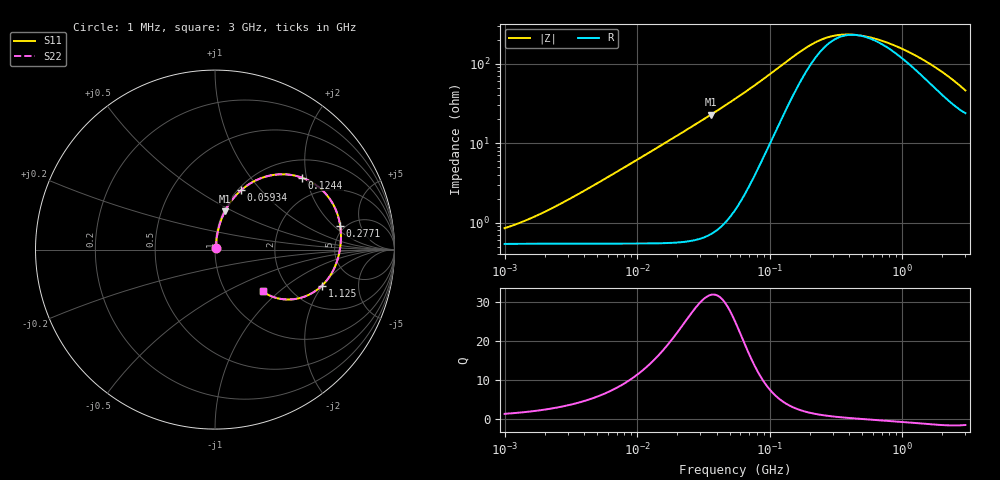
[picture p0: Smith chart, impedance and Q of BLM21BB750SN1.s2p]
! BLM21BB750SN1
# Hz S RI R 50
!Freq.(Hz) S11(Real) S11(Imag) S21(Real) S21(Imag) S12(Real) S12(Imag) S22(Real) S22(Imag)
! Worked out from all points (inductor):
!   401 points, 1 MHz to 3 GHz, reference 50 ohm
!   read as one part in series: L = 98.2 nH near 2.667 MHz
!   highest Q = 31.8 at 35.98 MHz (marker M1), where L = 101 nH
!   self-resonance near 452.7 MHz
!   S11 on the Smith chart (normalised r, x): 1 MHz: 1.01, +0.01; 59.34 MHz: 1.04, +0.78; 124.4 MHz: 1.42, +1.88; 277.1 MHz: 4.55, +2.43; 1.125 GHz: 2.97, -1.97; 3 GHz: 1.48, -0.79
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1000000  0.00541 0.00651  0.9946 -0.00651  0.9946 -0.00651  0.00541 0.00651
1786863  0.00552 0.0111  0.9945 -0.0111  0.9945 -0.0111  0.00552 0.0111
3823119  0.00595 0.0233  0.994 -0.0233  0.994 -0.0233  0.00595 0.0233
1.461624e7  0.0134 0.0884  0.9866 -0.0884  0.9866 -0.0884  0.0134 0.0884
2.362996e7  0.0265 0.1421  0.9735 -0.1421  0.9735 -0.1421  0.0265 0.1421
3.597591e7  0.0552 0.2132  0.9448 -0.2132  0.9448 -0.2132  0.0552 0.2132
5.477226e7  0.1237 0.3099  0.8763 -0.3099  0.8763 -0.3099  0.1237 0.3099
5.933785e7  0.1446 0.3299  0.8554 -0.3299  0.8554 -0.3299  0.1446 0.3299
7.248696e7  0.2118 0.3775  0.7882 -0.3775  0.7882 -0.3775  0.2118 0.3775
9.034013e7  0.3123 0.4138  0.6877 -0.4138  0.6877 -0.4138  0.3123 0.4138
1.244416e8  0.4853 0.4006  0.5147 -0.4006  0.5147 -0.4006  0.4853 0.4006
1.614254e8  0.6021 0.3268  0.3979 -0.3268  0.3979 -0.3268  0.6021 0.3268
2.094008e8  0.6695 0.2296  0.3305 -0.2296  0.3305 -0.2296  0.6695 0.2296
2.771263e8  0.6977 0.1325  0.3023 -0.1325  0.3023 -0.1325  0.6977 0.1325
3.523638e8  0.7018 0.0627  0.2982 -0.0627  0.2982 -0.0627  0.7018 0.0627
4.480278e8  0.6962 0.00245  0.3038 -0.00245  0.3038 -0.00245  0.6962 0.00245
5.929311e8  0.6809 -0.0616  0.3191 0.0616  0.3191 0.0616  0.6809 -0.0616
8.005644e8  0.6522 -0.1278  0.3478 0.1278  0.3478 0.1278  0.6522 -0.1278
1.125055e9  0.5964 -0.2004  0.4036 0.2004  0.4036 0.2004  0.5964 -0.2004
1.931433e9  0.4349 -0.2768  0.5651 0.2768  0.5651 0.2768  0.4349 -0.2768
2.407135e9  0.3486 -0.2711  0.6514 0.2711  0.6514 0.2711  0.3486 -0.2711
3e9  0.2664 -0.2334  0.7336 0.2334  0.7336 0.2334  0.2664 -0.2334
